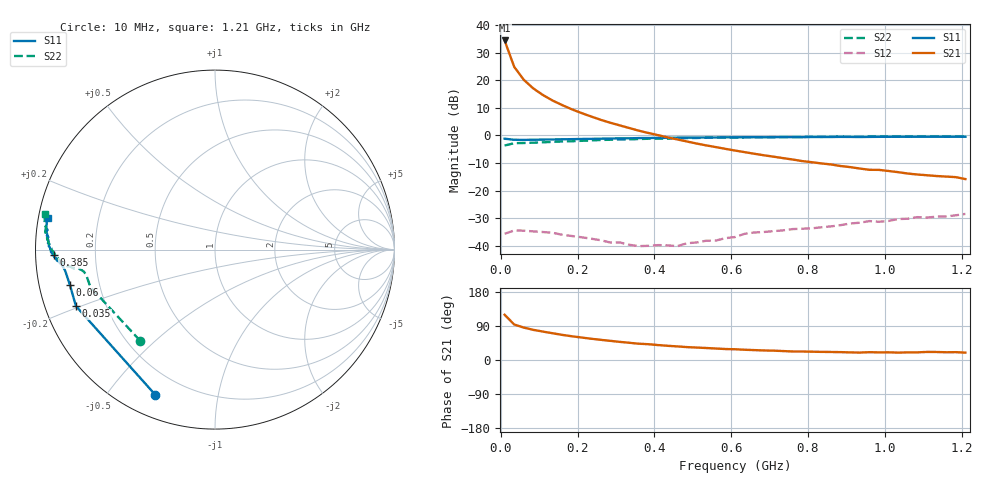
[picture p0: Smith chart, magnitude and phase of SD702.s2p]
!  POLYFET RF DEVICES
!  S PARAMETERS FOR
!  SD702 (EACH SIDE)
!  VDS=28, IDQ=400MA
! S1A2Die, Vds=28Vdc, Idq=400ma, Vgsth=2.63Vdc
! Date: Thu Jul 23 11:52:17 1998
# MHZ  S  MA  R  50.0000
! SCATTERING PARAMETERS :
! Freq=MHz Mag[s11] Ang[s11] Mag[s21] Ang[s21] Mag[s12] Ang[s12] Mag[s22] Ang[s22]
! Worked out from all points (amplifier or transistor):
!   49 points, 10 MHz to 1.21 GHz, reference 50 ohm
!   highest |S21| = 34.5 dB at 10 MHz (marker M1)
!   |S21| within 3 dB of that: start of sweep to 17.83 MHz
!   unconditionally stable (mu >= 1): 254.1 MHz to end of sweep
!   at 210 MHz: K = 0.77, MSG = 22.5 dB, |S12| = -36.9 dB
!   at 610 MHz: K = 1.65, MAG = 11.0 dB, |S12| = -36.8 dB
!   at 1.21 GHz: K = 1.10, MAG = 4.4 dB, |S12| = -28.4 dB
!   S11 on the Smith chart (normalised r, x): 10 MHz: 0.10, -0.67; 35 MHz: 0.09, -0.19; 60 MHz: 0.09, -0.12; 385 MHz: 0.05, -0.02; 1.21 GHz: 0.03, +0.09
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10  0.8744 -112.4  52.93 119.3  0.01651 29.2  0.6571 -129.4
35  0.8363 -157.9  17.56 93.7  0.01893 8.9  0.7248 -163.3
60  0.8321 -166.4  10.22 85.5  0.01877 2.6  0.731 -168.7
85  0.8379 -170.0  7.113 79.5  0.01821 0.6  0.7404 -170.4
110  0.8422 -171.7  5.408 75.0  0.01774 -0.4  0.7515 -171.3
135  0.8467 -172.7  4.304 70.6  0.01721 -4.0  0.7658 -172.0
160  0.8535 -173.7  3.557 66.3  0.01582 -2.4  0.7795 -172.1
185  0.858 -174.3  2.986 62.6  0.01502 -3.7  0.7859 -172.4
210  0.8648 -174.8  2.555 59.4  0.01428 -1.8  0.801 -172.7
235  0.8691 -175.2  2.215 56.2  0.01345 1.1  0.8137 -173.4
260  0.8748 -175.7  1.928 53.3  0.01261 4.9  0.8289 -173.6
285  0.8823 -176.0  1.706 50.5  0.01146 7.6  0.8368 -174.0
335  0.8887 -177.1  1.363 45.4  0.0104 12.4  0.8502 -175.2
385  0.8999 -178.0  1.109 41.7  0.00998 23.6  0.8731 -176.4
410  0.9054 -178.4  1.013 39.4  0.01028 35.0  0.8787 -177.3
460  0.9137 -179.1  0.8481 35.9  0.00983 37.8  0.8908 -177.9
485  0.9143 -179.6  0.7782 34.0  0.01113 49.0  0.8976 -179.0
610  0.925 178.3  0.5332 28.4  0.01439 72.4  0.9202 178.5
660  0.9315 177.8  0.4666 26.1  0.0174 74.5  0.9307 177.5
810  0.9402 175.3  0.3279 21.9  0.02071 79.9  0.9458 174.6
1010  0.9468 172.5  0.2269 20.3  0.02822 88.1  0.9637 171.5
1210  0.9479 169.3  0.1621 19.5  0.03783 84.6  0.9659 168.2
